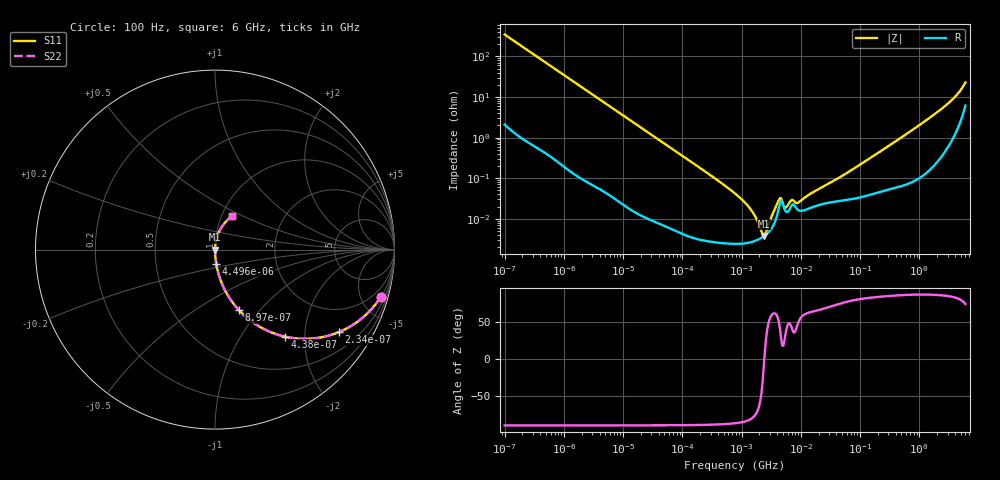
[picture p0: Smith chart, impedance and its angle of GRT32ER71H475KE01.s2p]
!Murata Part Number: GRT32ER71H475KE01
!These Parameters are Measured in Series Mode Connection
!Data Generated on Jun 19, 2026
!  o--ll--o
!Port1  Port2
!  o------o
!Operation Temp=25[degC], DC Bias Voltage=0[V]
!Freq. Start=100[Hz] Stop=6[GHz] 401[Steps]
# Hz S RI R 50
!Freq.(Hz) S11(Real) S11(Imag) S21(Real) S21(Imag) S12(Real) S12(Imag) S22(Real) S22(Imag)
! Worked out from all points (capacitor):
!   401 points, 100 Hz to 6 GHz, reference 50 ohm
!   read as one part in series: C = 4.56 uF near 109 Hz
!   lowest |Z| = 3.76 mohm at 2.373 MHz (marker M1)
!   series resonance near 2.423 MHz, so ESL is about 950 pH
!   S11 on the Smith chart (normalised r, x): 100 Hz: 1.04, -6.97; 234 Hz: 1.02, -2.98; 438 Hz: 1.01, -1.60; 897 Hz: 1.00, -0.78; 4.496 kHz: 1.00, -0.16; 6 GHz: 1.12, +0.44
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100  0.9226 -0.2643  0.0774 0.2643  0.0774 0.2643  0.9226 -0.2643
234  0.689 -0.4602  0.311 0.4602  0.311 0.4602  0.689 -0.4602
438  0.3901 -0.4849  0.6099 0.4849  0.6099 0.4849  0.3901 -0.4849
897  0.1342 -0.3381  0.8658 0.3381  0.8658 0.3381  0.1342 -0.3381
2008  0.0306 -0.1697  0.9694 0.1697  0.9694 0.1697  0.0306 -0.1697
4496  0.0066 -0.0779  0.9934 0.0779  0.9934 0.0779  0.0066 -0.0779
40335  0.000154 -0.00881  0.9998 0.00881  0.9998 0.00881  0.000154 -0.00881
774597  2.42e-05 -0.000419  1 0.000419  1 0.000419  2.42e-05 -0.000419
1212075  2.52e-05 -0.000226  1 0.000226  1 0.000226  2.52e-05 -0.000226
1813585  2.97e-05 -9.03e-05  1 9.03e-05  1 9.03e-05  2.97e-05 -9.03e-05
2372521  3.7e-05 -6.6e-06  1 6.6e-06  1 6.6e-06  3.7e-05 -6.6e-06
3103719  5.41e-05 8.47e-05  0.9999 -8.47e-05  0.9999 -8.47e-05  5.41e-05 8.47e-05
4440638  0.000243 0.000211  0.9998 -0.000211  0.9998 -0.000211  0.000243 0.000211
5554849  0.000152 0.000108  0.9998 -0.000108  0.9998 -0.000108  0.000152 0.000108
6948629  0.00021 0.000199  0.9998 -0.000199  0.9998 -0.000199  0.00021 0.000199
9090158  0.000163 0.000191  0.9998 -0.000191  0.9998 -0.000191  0.000163 0.000191
1.555665e7  0.000193 0.000395  0.9998 -0.000395  0.9998 -0.000395  0.000193 0.000395
5.211241e7  0.000284 0.00115  0.9997 -0.00115  0.9997 -0.00115  0.000284 0.00115
3.124326e8  0.00057 0.00638  0.9994 -0.00638  0.9994 -0.00638  0.00057 0.00638
2.450438e9  0.00639 0.0525  0.9936 -0.0525  0.9936 -0.0525  0.00639 0.0525
4.009986e9  0.0216 0.0975  0.9784 -0.0975  0.9784 -0.0975  0.0216 0.0975
6e9  0.0967 0.1873  0.9033 -0.1873  0.9033 -0.1873  0.0967 0.1873
